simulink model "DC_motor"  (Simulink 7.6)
settings: Solver=ode23tb  StartTime=0.0  StopTime=3  RelTol=1e-3
StopFcn:
  | close all
  | load DC_motor.mat
  | plotyy(x(1,:),x(2,:),x(1,:),x(3,:))
  | %axis([0 3 0 1200])
  | grid
  | title('Courant aux armatures et vitesse du moteur')
  | xlabel('temps')
libraries: powerlib x4, electricdrivelib x1

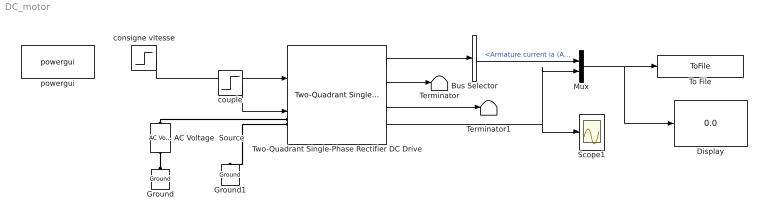
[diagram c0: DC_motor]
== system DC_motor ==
  AC Voltage  Source : powerlib/Electrical Sources/AC Voltage Source  DialogController=POWERSYS.PowerSysDialog  SystemSampleTime=-1  Amplitude=220  Phase=0  Frequency=60  SampleTime=0  Measurements=None
  Bus Selector : BusSelector  OutputSignals=Armature current ia (A)
  Display : Display
  Ground : powerlib/Elements/Ground  DialogController=POWERSYS.PowerSysDialog  PhysicalDomain=powersysdomain  SubClassName=unknown  LeftPortType=p1  RightPortType=p1  LConnTagsString=a
  Ground1 : powerlib/Elements/Ground  DialogController=POWERSYS.PowerSysDialog  PhysicalDomain=powersysdomain  SubClassName=unknown  LeftPortType=p1  RightPortType=p1  LConnTagsString=a
  Mux : Mux  Inputs=2
  Scope1 : Scope
  Terminator : Terminator
  Terminator1 : Terminator
  To File : ToFile  Filename=DC_motor  MatrixName=x
  Two-Quadrant Single-Phase Rectifier DC Drive : electricdrivelib/DC drives/Two-Quadrant Single-Phase Rectifier DC Drive  SystemSampleTime=-1  showMaskWarnings=on  AverageValue=off  MechanicalLoad=Torque Tm  driveType=DC1
  consigne vitesse : Step  Time=0  After=1000  SampleTime=0
  couple : Step  Time=0  After=20  SampleTime=0
  powergui : powerlib/powergui  SystemSampleTime=-1  SimulationMode=Discrete  SampleTime=1e-4  frequency=60  SPID=off  DisableSnubberDevices=off  DisableRonSwitches=off  DisableVfSwitches=off  SwTol=0  Interpol=off  frequencyindice=0  echomessages=off  HookPort=off  DisplayEquations=off  FunctionMessages=off  EnableUseOfTLC=off  x0status=blocks  RestoreLinks=warning  ResistiveCurrentMeasurement=off  Frange=[0:2:500]  Ylog=off  Xlog=on  ShowGrid=off  save=off  variable=ZData  ZoomFFT=on  StartTime=0.0  cycles=1  DisplayStyle=1  fundamental=60  FreqAxis=off  MaxFrequency=1000  frequencyindicesteady=1  RmsSteady=1  display=off  Ts=0  methode=off
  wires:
  consigne vitesse/1 -> Two-Quadrant Single-Phase Rectifier DC Drive/1
  couple/1 -> Two-Quadrant Single-Phase Rectifier DC Drive/2
  Two-Quadrant Single-Phase Rectifier DC Drive/1 -> Bus Selector/1
  Mux/1 -> To File/1, Display/1
  Two-Quadrant Single-Phase Rectifier DC Drive/4 -> Scope1/1, Mux/2
  Bus Selector/1 -> Mux/1  "<Armature current ia (A)>"
  Two-Quadrant Single-Phase Rectifier DC Drive/2 -> Terminator/1
  Two-Quadrant Single-Phase Rectifier DC Drive/3 -> Terminator1/1
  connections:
  AC Voltage  Source/LConn1 -- Ground/LConn1
  AC Voltage  Source/RConn1 -- Two-Quadrant Single-Phase Rectifier DC Drive/LConn1
  Two-Quadrant Single-Phase Rectifier DC Drive/LConn2 -- Ground1/LConn1
